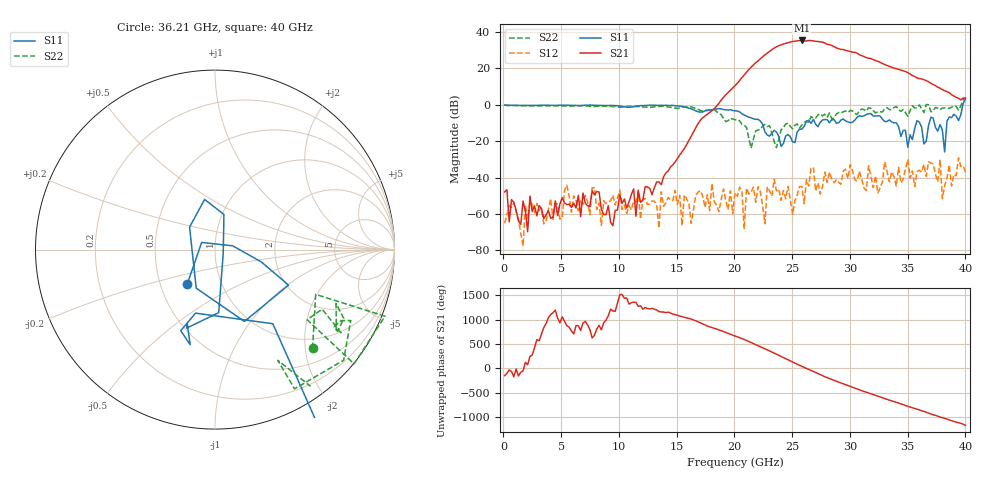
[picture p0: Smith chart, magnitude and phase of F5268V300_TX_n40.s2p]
!S2P File: Measurements: S11,S21,S12,S22
# MHz S  RI  R 50
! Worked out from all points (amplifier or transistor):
!   201 points, 100 MHz to 40 GHz, reference 50 ohm
!   highest |S21| = 35.4 dB at 25.84 GHz (marker M1)
!   |S21| within 3 dB of that: 23.81 GHz to 28.5 GHz (4.687 GHz wide, 17.9 % of centre)
!   unconditionally stable (mu >= 1): start of sweep to 26.22 GHz; 33.25 GHz to 35.39 GHz; 36.88 GHz to 39.6 GHz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
!   at 6.684 GHz: K = 2437.76, MAG = -41.6 dB, |S12| = -52.2 dB
!   at 20.05 GHz: K = 17.88, MAG = 13.9 dB, |S12| = -48.4 dB
!   at 40 GHz: K = 39.98, MSG = 20.3 dB, |S12| = -36.9 dB
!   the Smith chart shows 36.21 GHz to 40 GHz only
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100  -0.9851 0.0469  -0.00349 -0.00201  -0.00037 -0.000412  -0.9774 0.0381
6883  0.0934 0.9632  -0.00335 -0.00167  0.000744 -0.00167  -0.487 0.8052
13467  0.8968 -0.3432  0.000799 0.00755  0.000404 5.44e-05  0.8382 0.3323
20050  -0.3867 -0.5635  1.828 -2.835  0.00332 -0.00188  -0.1608 -0.3509
21646  -0.4114 0.00443  -10.59 6.684  -0.00308 0.00451  -0.0798 -0.0811
22444  -0.2504 0.1526  9.672 18.59  -0.0016 -0.00041  -0.2175 -0.1476
23242  -0.1361 0.0976  29.51 -14.39  -0.00279 -0.00136  -0.1061 -0.1293
23841  0.0685 0.1187  -4.546 -41.83  -0.00154 -0.00452  -0.1121 0.02
24639  0.0897 0.1228  -50.57 6.204  0.00217 0.0053  -0.2456 0.1953
25237  0.0877 -0.027  -15.56 54.07  0.00176 -0.00147  -0.2166 0.1682
25836  0.1461 -0.1554  44.93 37.97  -0.00536 0.00187  -0.1115 0.2547
26434  0.2483 -0.2804  53.39 -23.16  0.00572 0.00131  -0.0388 0.329
26833  0.2819 -0.2813  22.22 -52.46  -0.015 -0.0117  0.065 0.4257
27232  0.1244 -0.2177  -17.8 -52.05  0.00294 0.00652  0.0483 0.5228
27631  0.0209 -0.3842  -46.8 -25.14  0.00319 0.00475  0.2329 0.4411
28629  -0.1092 -0.3774  -14.93 36.69  0.00706 0.00136  0.3339 0.2872
29626  -0.1653 -0.3182  28.64 13.13  -0.00352 -0.0165  0.399 0.5493
30624  -0.3237 -0.3199  10.62 -24.08  -0.000417 -0.00794  0.518 0.1557
31821  -0.5241 -0.2302  -17.91 -5.351  -0.00572 0.00925  0.7527 0.269
33417  -0.3827 0.0122  4.575 10.47  -0.000764 0.00752  0.6423 -0.3716
35013  -0.0526 -0.0433  3.852 -6.623  -0.00771 0.0304  0.4551 -0.1693
40000  0.3424 -1.387  -0.0679 -1.524  -0.00608 0.0129  0.8492 -1.364
